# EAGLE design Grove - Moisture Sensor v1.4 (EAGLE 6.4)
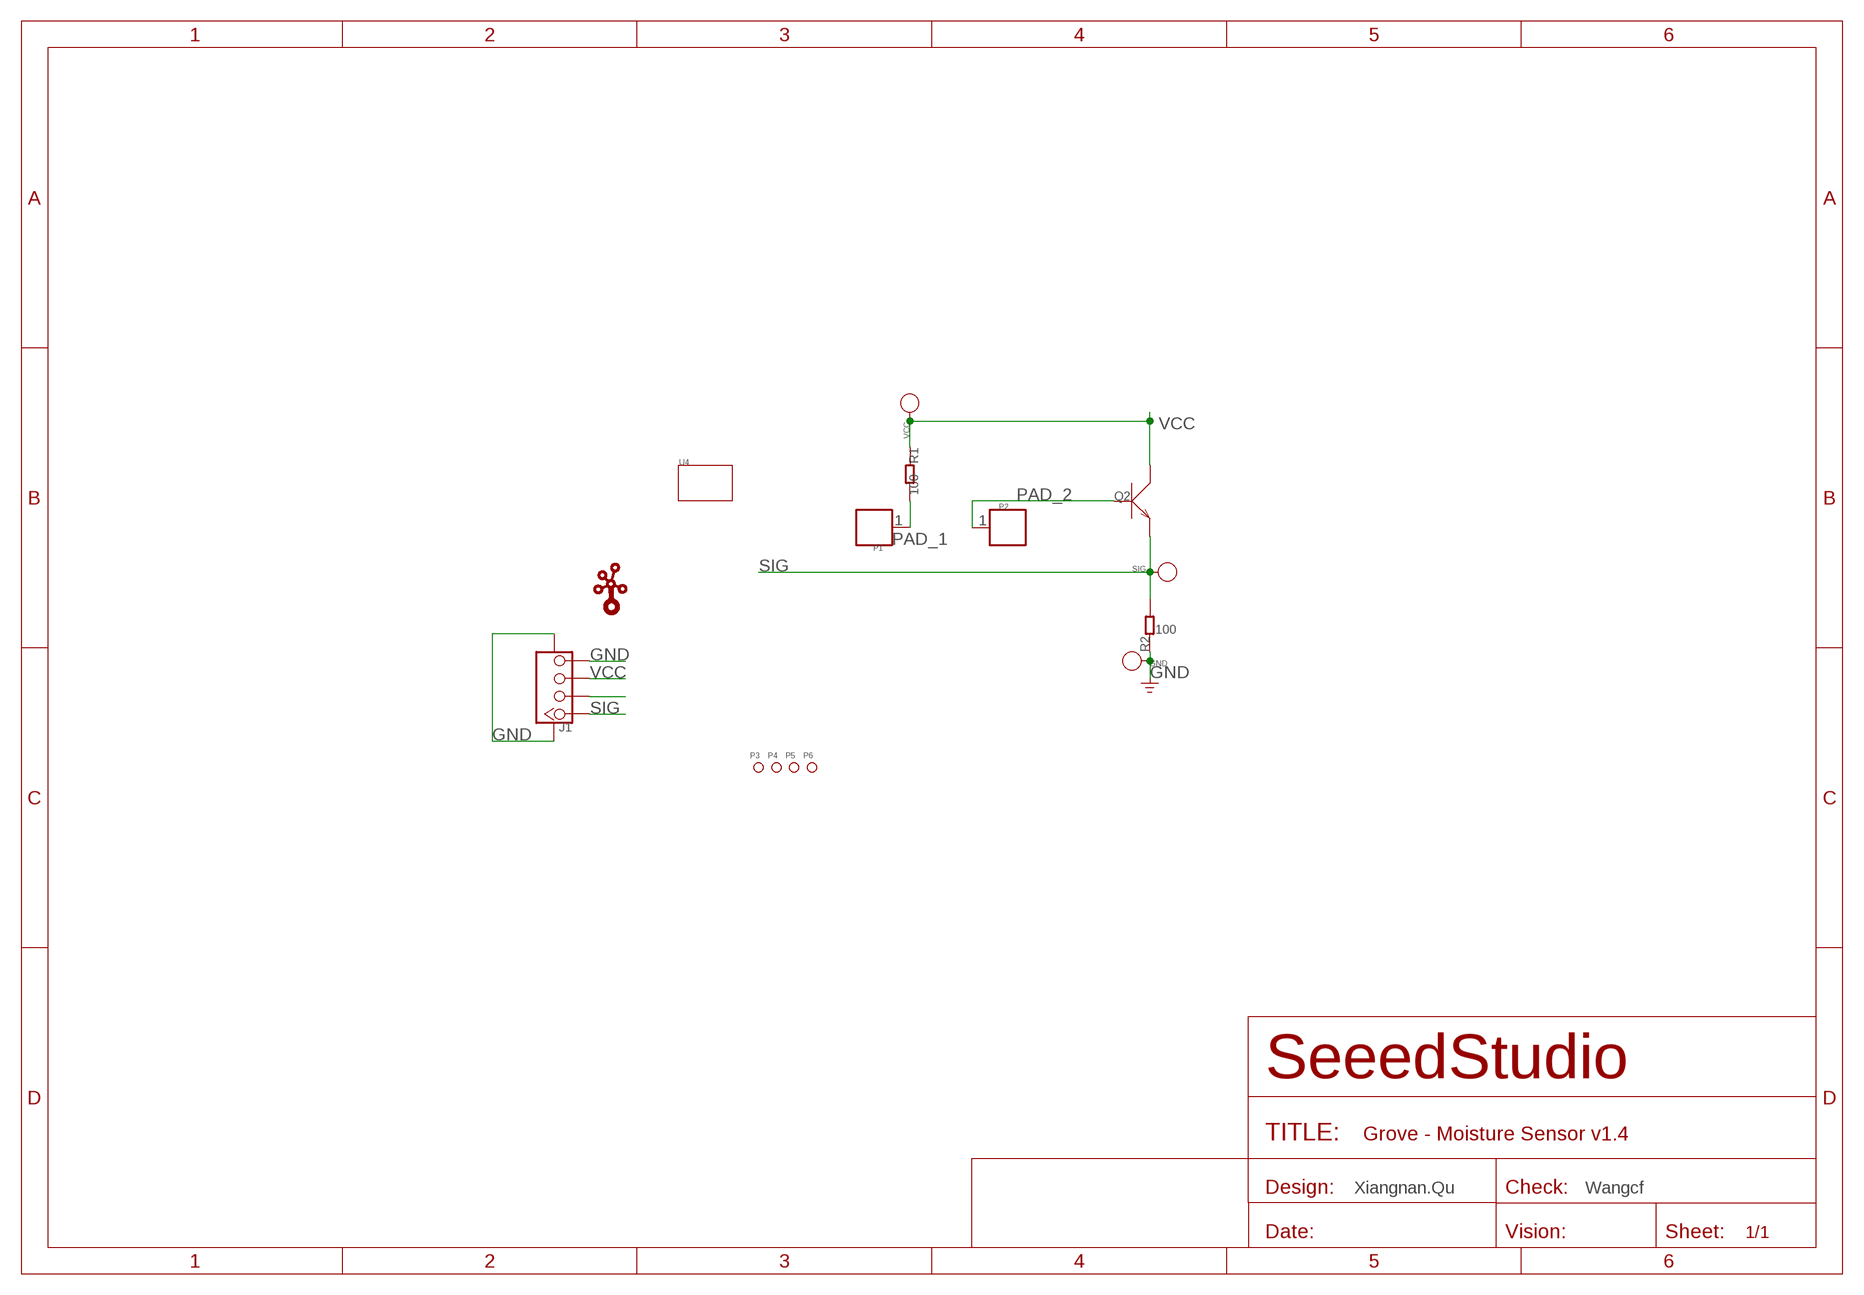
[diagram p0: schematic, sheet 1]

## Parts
GND  PAD-TEST-POINT'4545'  [TP_4545]
J1  TWIG-4P-2.0-SMD-FEMALE-REINFORCE'90D'  [4P-SMD-2.0-90D]
P1  PAD.03  [1P-SMD-0.76X0.76]
P2  PAD.03  [1P-SMD-0.76X0.76]
P3  PAD-MARK'ANNULAR'  [ROUND-MARK-1.0]
P4  PAD-MARK'ANNULAR'  [ROUND-MARK-1.0]
P5  PAD-MARK'ANNULAR'  [ROUND-MARK-1.0]
P6  PAD-MARK'ANNULAR'  [ROUND-MARK-1.0]
Q2  TRANSISTOR-NPN-SOT23  [SOT23]
R1  100  R-0603  [R0603]
R2  100  R-0603  [R0603]
SIG  PAD-TEST-POINT'4545'  [TP_4545]
U4  MODULE_TWIGSPECIAL  [MODULE_3U-DIM-W/-DRILL-SPECIAL]
U$1  LOGO-TWIG  [TWIGLOGO]
VCC  PAD-TEST-POINT'4545'  [TP_4545]

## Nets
GND: GND.T J1.4 J1.SS1 J1.SS2 R2.1
N$4: J1.2
PAD_1: P1.1 R1.2
PAD_2: P2.1 Q2.1(B)
SIG: J1.1 Q2.2(E) R2.2 SIG.T
VCC: J1.3 Q2.3(C) R1.1 VCC.T

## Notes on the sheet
- Xiangnan.Qu | Wangcf

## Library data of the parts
GND SIG VCC = Discrete:PAD-TEST-POINT; PARTNO: DNP
J1 = Connector:TWIG-4P-2.0-SMD-FEMALE-REINFORCE
P1 P2 = Discrete:PAD
P3-P6 = Discrete:PAD-MARK; PARTNO: DNP
Q2 = Discrete:TRANSISTOR-NPN*: NPN audion
R1 R2 = Discrete:R*
U4 = Grove_-_Moisture_Sensor_v1.4:MODULE_TWIG
U$1 = Logo:LOGO-TWIG; PARTNO: DNP

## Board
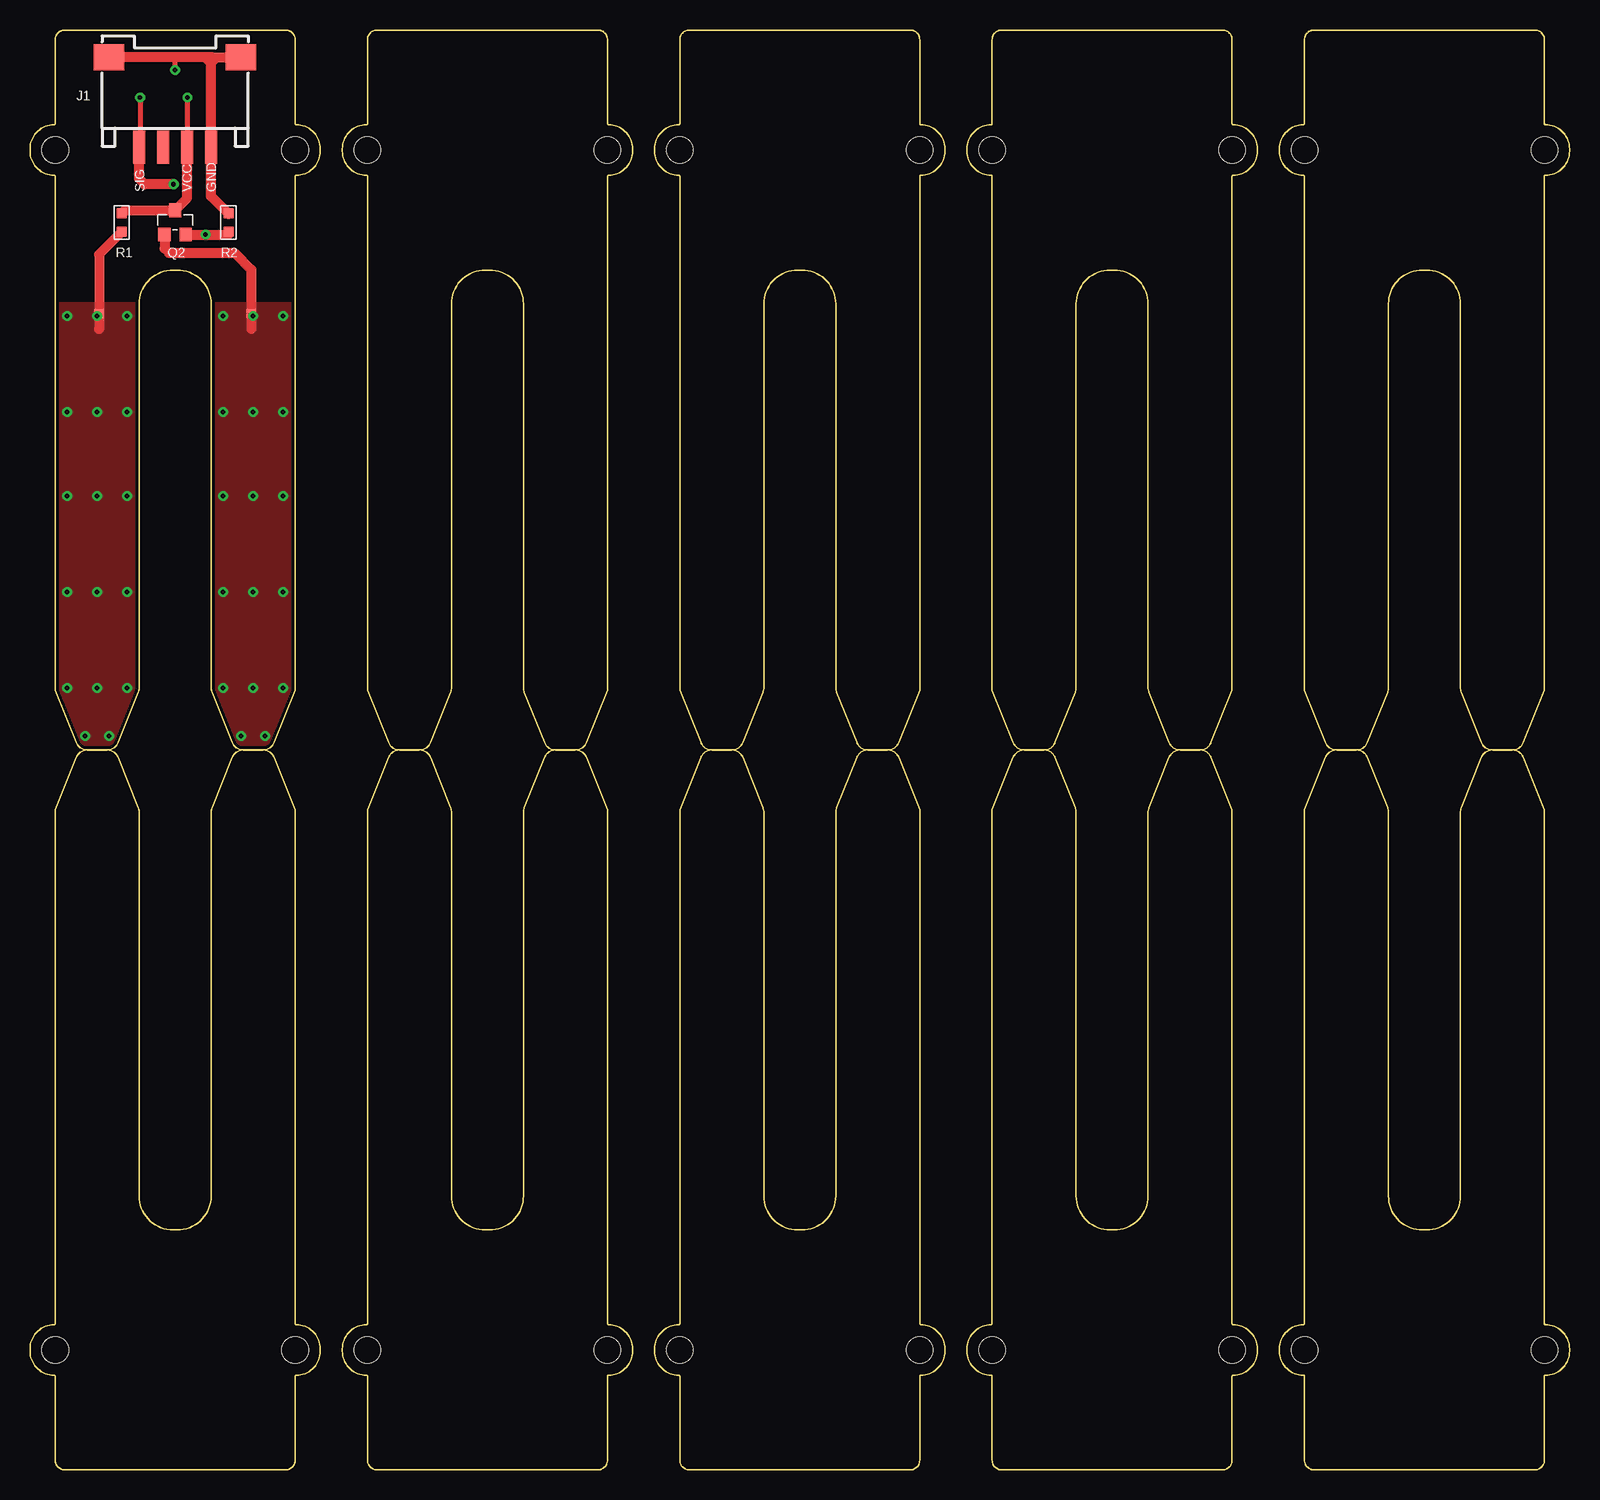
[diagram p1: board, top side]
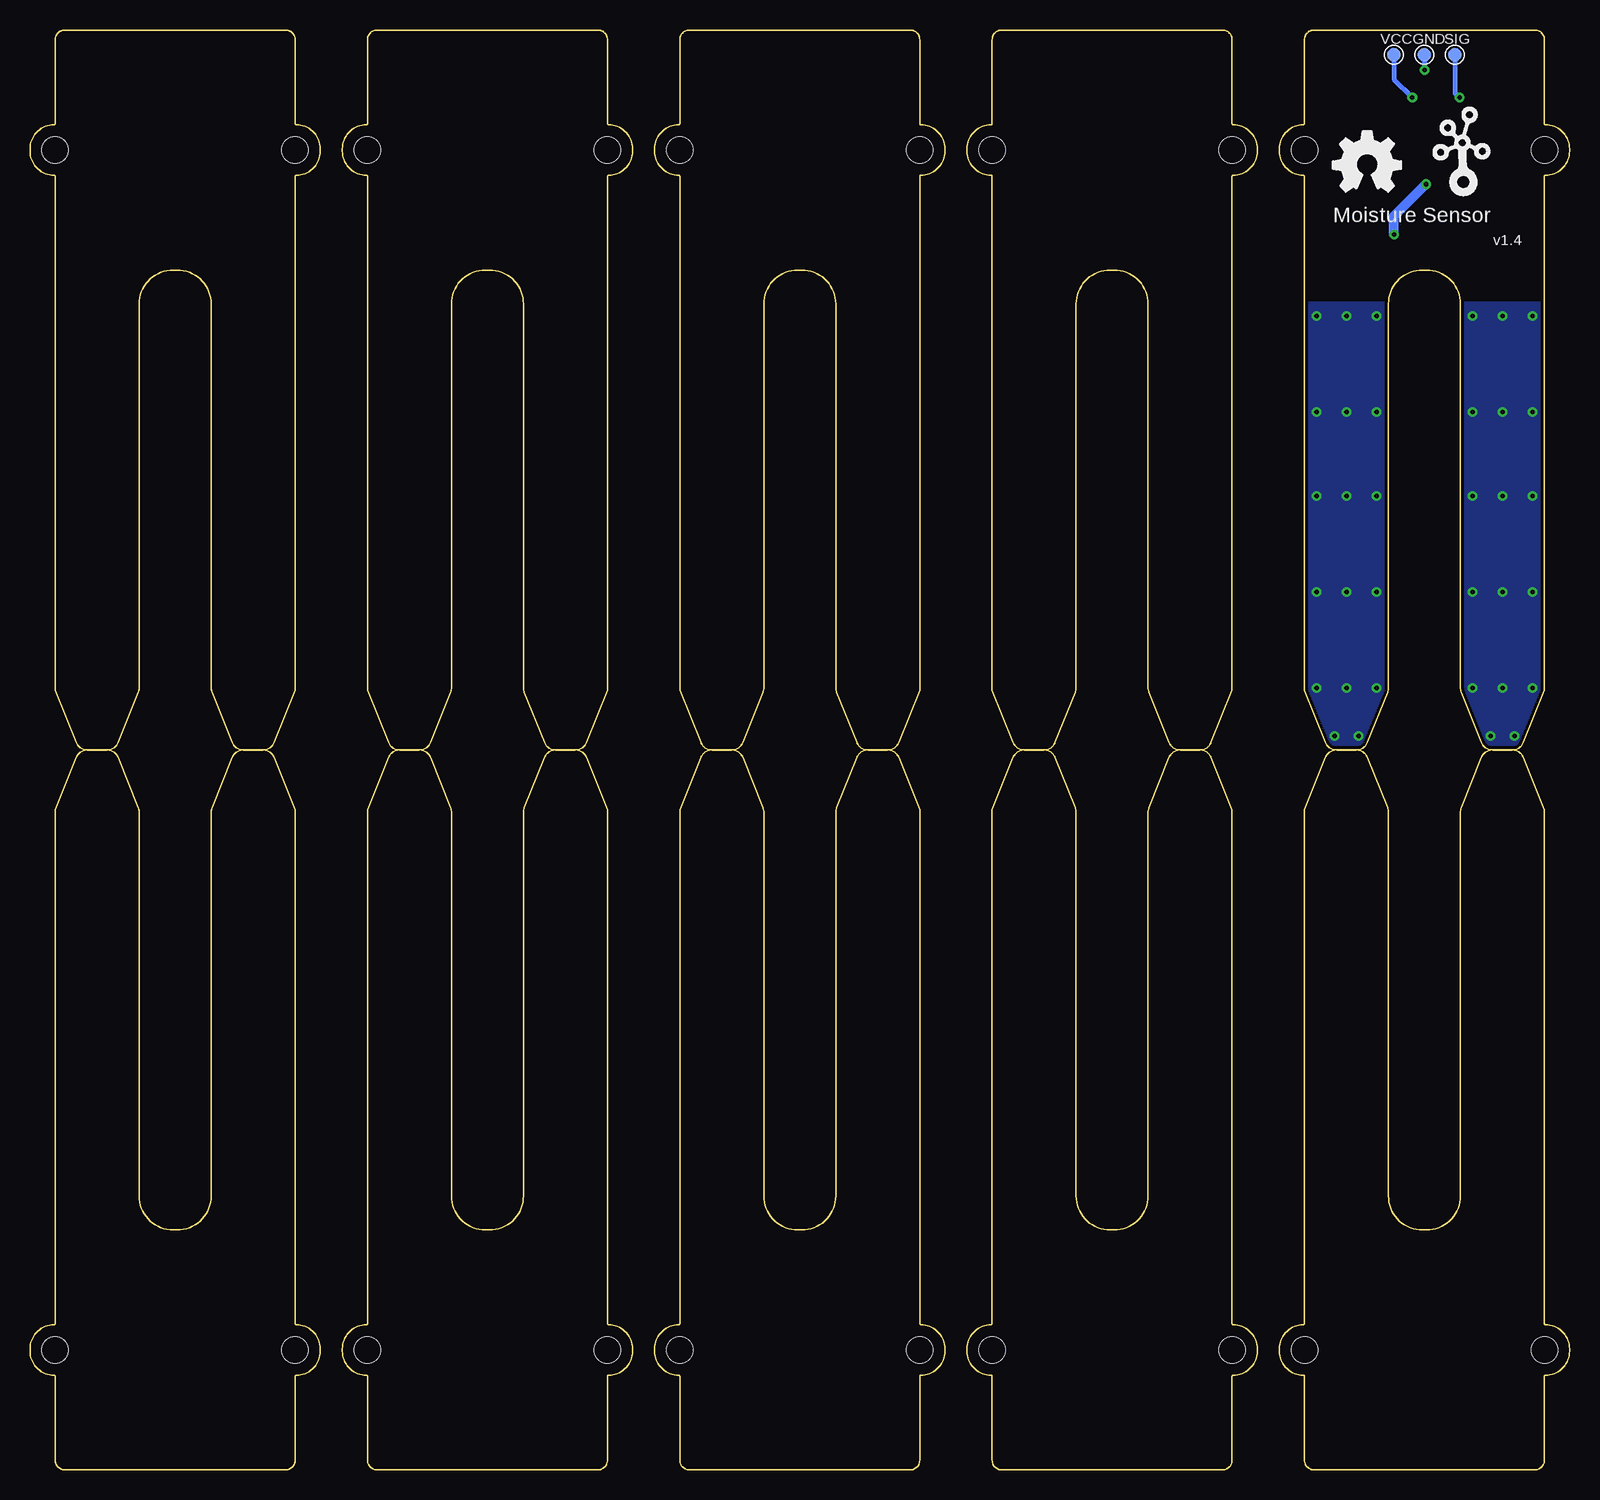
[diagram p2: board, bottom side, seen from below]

Size 128.34 x 119.99 mm. Coordinates in mm from the lower left corner, seen from the top.
Copper layers (1*16): Top 0.035mm / dielectric 1.5mm / Bottom 0.035mm
Design rules "SeeedStudio_rule_no_angle_090911 *": minimum track width 6mil, minimum drill 12mil, track to track 6mil, track to pad 6mil, pad to pad 6mil, via to via 6mil, smd to smd 0mil, copper to edge 10mil, drill to drill 10mil, minimum pad ring 10mil, minimum via ring 6mil, stop-mask expansion 2mil, vias tented up to drill 25mil, thermal gap 10mil
Holes 2.03 mm at 7.65,124.28 120.68,124.28 120.68,-4.62 7.65,-4.62

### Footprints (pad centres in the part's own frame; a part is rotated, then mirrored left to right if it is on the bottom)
TP_4545 = smd 1.143 x 1.143: T 0,0
4P-SMD-2.0-90D = smd 1.01 x 2.74: 1 -3,-0.1; 2 -1,-0.1; 3 1,-0.1; 4 3,-0.1 | smd 2.54 x 2.184: SS1 -5.5,7.4; SS2 5.5,7.4
1P-SMD-0.76X0.76 = smd 0.762 x 0.762: 1 0,0
ROUND-MARK-1.0 = smd 1.016 x 1.016: P$1 0,0
SOT23 = smd 1.016 x 1.143: 1 -0.889,-1.016; 2 0.889,-1.016; 3 0,1.016
R0603 = smd 0.889 x 0.889: 1 -0.762,0; 2 0.762,0
MODULE_3U-DIM-W/-DRILL-SPECIAL = hole 2.2: 10,20; -10,20

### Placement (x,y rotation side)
GND  12.1,117.93 0 bottom
J1  12.1,110.31 0 top
P1  5.75,96.34 0 top
P2  18.45,96.34 0 top
P3  not placed on the board
P4  not placed on the board
P5  not placed on the board
P6  not placed on the board
Q2  12.1,103.96 0 top
R1  7.65,103.96 270 top
R2  16.55,103.96 270 top
SIG  9.56,117.93 0 bottom
U1  [MODULE_3U-DIM-W/-DRILL-SPECIAL]  12.1,89.99 0 top
U2  [MODULE_3U-DIM-W/-DRILL-SPECIAL]  12.1,30 180 top
U3  [MODULE_3U-DIM-W/-DRILL-SPECIAL]  38.13,89.99 0 top
U4  38.13,30 180 top
U5  [MODULE_3U-DIM-W/-DRILL-SPECIAL]  64.17,89.99 0 top
U6  [MODULE_3U-DIM-W/-DRILL-SPECIAL]  64.17,30 180 top
U7  [MODULE_3U-DIM-W/-DRILL-SPECIAL]  90.2,89.99 0 top
U8  [MODULE_3U-DIM-W/-DRILL-SPECIAL]  90.2,30 180 top
U9  [MODULE_3U-DIM-W/-DRILL-SPECIAL]  116.24,89.99 0 top
U10  [MODULE_3U-DIM-W/-DRILL-SPECIAL]  116.24,30 180 top
U$1  8.91,107.12 0 bottom
U$2  [OSHW_FILLX200_NOTEXT]  19.72,106.5 0 bottom
VCC  14.64,117.93 0 bottom

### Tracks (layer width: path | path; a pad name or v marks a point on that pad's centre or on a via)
GND  (via drill 0.38 pad 0.81)
  Top 0.406: v12.1,116.66 12.1,117.71
  Top 0.813: R2.1 16.55,104.68 15.1,106.12 J1.4 15.1,117.22 | 15.27,117.71 12.1,117.71 J1.SS1 | 15.27,117.71 J1.SS2 | 15.1,117.25 15.1,117.54 15.27,117.71 | 15.1,117.22 14.64,117.68 | 15.1,117.22 15.1,117.25 | 15.1,117.25 15.53,117.68
  Bottom 0.406: GND.T v12.1,116.66
PAD_1  (via drill 0.38 pad 0.81)
  Top 0.813: 5.75,95.07 P1.1 5.75,101.3 R1.2
  other vias: 4.6,61.15 6.6,61.15 3.1,96.15 5.6,96.15 8.1,96.15 5.6,88.15 8.1,88.15 8.1,81.15 5.6,81.15 3.1,65.15 3.1,73.15 3.1,81.15 3.1,88.15 5.6,73.15 8.1,73.15 5.6,65.15 8.1,65.15
  pour Top (no thermals): 2.1,97.15 9.1,97.15 9.1,60.15 2.1,60.15
  pour Bottom (no thermals): 2.1,97.15 9.1,97.15 9.1,60.15 2.1,60.15
PAD_2  (via drill 0.38 pad 0.81)
  Top 0.813: 18.45,95.07 P2.1 18.45,100.03 17.05,101.42 11.59,101.42 11.21,101.81 Q2.1
  other vias: 17.6,61.15 19.6,61.15 16.1,65.15 18.6,65.15 21.1,65.15 16.1,96.15 18.6,96.15 21.1,96.15 16.1,88.15 18.6,88.15 21.1,88.15 16.1,81.15 18.6,81.15 21.1,81.15 16.1,73.15 18.6,73.15 21.1,73.15
  pour Top (no thermals): 15.1,97.15 22.1,97.15 22.1,60.15 15.1,60.15
  pour Bottom (no thermals): 15.1,97.15 22.1,97.15 22.1,60.15 15.1,60.15
SIG  (via drill 0.38 pad 0.81)
  Top 0.406: v9.18,114.38 9.18,110.29 J1.1
  Top 0.813: Q2.2 v14.64,102.95 16.55,102.95 R2.2 | J1.1 9.1,107.6 9.56,107.14 v11.97,107.14
  Bottom 0.406: SIG.T 9.56,114.76 v9.18,114.38
  Bottom 0.813: v14.64,102.95 14.64,104.47 v11.97,107.14
VCC  (via drill 0.38 pad 0.81)
  Top 0.406: v13.12,114.38 13.12,110.08 13.1,110.06
  Top 0.813: J1.3 13.1,110.06 13.1,105.98 Q2.3 7.91,104.98 R1.1
  Bottom 0.406: VCC.T 14.64,115.9 v13.12,114.38

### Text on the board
tPlace: SIG | VCC | GND
bPlace: Moisture Sensor | v1.4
